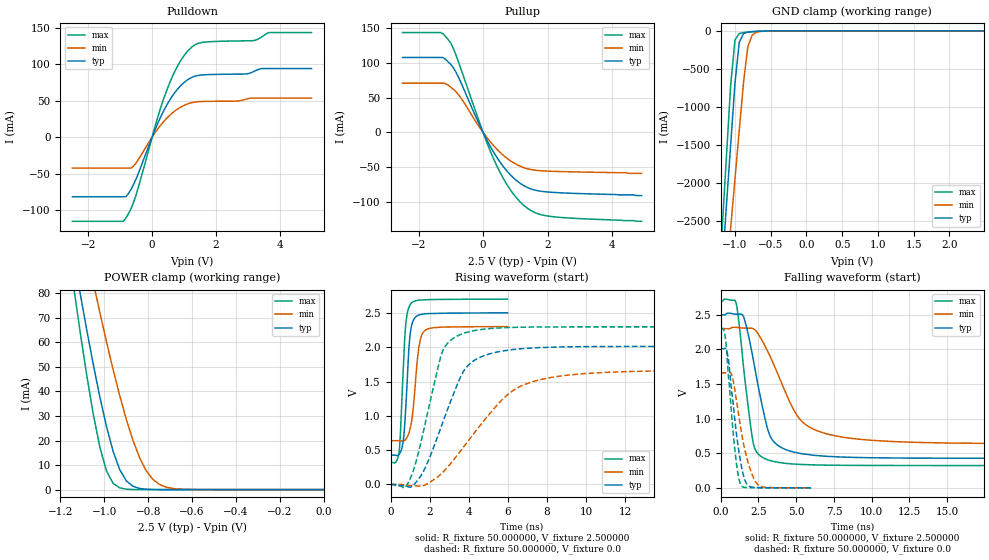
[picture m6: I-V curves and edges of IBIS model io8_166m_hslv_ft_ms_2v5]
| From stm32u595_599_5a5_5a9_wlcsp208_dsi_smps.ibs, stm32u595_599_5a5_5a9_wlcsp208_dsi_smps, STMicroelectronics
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|   Model io8_166m_hslv_ft_ms_2v5
[Model]  io8_166m_hslv_ft_ms_2v5
Model_type I/O
Polarity   Non-Inverting
Enable   Active-Low
Vinl =   0.750000V
Vinh =   1.750000V
Vmeas =  1.250000V
Cref =   50.000000pF
Rref =   100.000000M
Vref =   0.0V
C_comp   3.458600pF   3.458000pF   3.495600pF
[Temperature Range]   25.000000   0.140000k   -40.000000
[Pullup Reference]   2.500000V   2.300000V   2.700000V
[Pulldown Reference]   0.0V   0.0V   0.0V
[POWER Clamp Reference]   2.500000V   2.300000V   2.700000V
[GND Clamp Reference]   0.0V   0.0V   0.0V
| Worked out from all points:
|   slope of the pulldown table from 0 to 0.375 V, typ, clamps not added: 10.1 ohm
|   slope of the pullup table from 0 to 0.375 V, typ, clamps not added: 11.7 ohm
|   GND clamp passes 1 mA (typ) near -0.50 V on its own axis
|   POWER clamp passes 1 mA (typ) near -0.86 V on its own axis
|   rising waveform, R_fixture 50.000000, V_fixture 2.500000: 20-80 % time 251ps typ, 332ps min, 234ps max; typ from 0.428 V to 2.5 V
|   rising waveform, R_fixture 50.000000, V_fixture 0.0: 20-80 % time 1.64ns typ, 2.93ns min, 1.12ns max; typ from 0 V to 2.01 V
|   falling waveform, R_fixture 50.000000, V_fixture 2.500000: 20-80 % time 1.17ns typ, 2.21ns min, 750ps max; typ from 2.5 V to 0.428 V
|   falling waveform, R_fixture 50.000000, V_fixture 0.0: 20-80 % time 665ps typ, 867ps min, 543ps max; typ from 2.01 V to 0 V
[Pulldown]
|Voltage   I(typ)   I(min)   I(max)
-2.5V     -81.62mA   -42.31mA   -115.3mA
-900mV    -81.62mA   -42.31mA   -115.3mA
-820mV    -81.43mA   -42.31mA   -110.6mA
-500mV    -56.95mA   -35.08mA   -78.57mA
140mV     15.18mA    9.02mA     22.02mA
460mV     44mA       25.98mA    64.38mA
860mV     68.91mA    40.27mA    102.2mA
1.26V     82.21mA    47.42mA    124mA
1.66V     85.54mA    49mA       130.3mA
3.18V     89.84mA    53.64mA    132.3mA
3.66V     94.01mA    53.64mA    143.3mA
5V        94.01mA    53.64mA    143.3mA
[Pullup]
|Voltage   I(typ)   I(min)   I(max)
-2.5V     108.1mA    71.02mA    143.9mA
-1.32V    108.1mA    71.02mA    143.9mA
-1.24V    107.8mA    71.02mA    142.1mA
-1V       97.95mA    65.11mA    128.6mA
-680mV    71.17mA    49.12mA    90.46mA
-40mV     3.893mA    2.628mA    5.181mA
360mV     -30.97mA   -20.78mA   -41.56mA
840mV     -60.71mA   -40.52mA   -82.21mA
1.32V     -78.06mA   -51.54mA   -107.3mA
1.64V     -83.42mA   -54.54mA   -116.1mA
2.12V     -86.16mA   -55.91mA   -121.1mA
4.92V     -91mA      -59mA      -128mA
[GND_clamp]
|Voltage   I(typ)   I(min)   I(max)
-2.5V     -9.641A    -9.693A    -9.352A
-1.18V    -3.114A    -3.874A    -2.614A
-1.12V    -2.301A    -3.23A     -1.656A
-1.06V    -1.489A    -2.587A    -706.2mA
-1V       -685.8mA   -1.945A    -119.3mA
-940mV    -149.7mA   -1.304A    -34.73mA
-880mV    -35.54mA   -672.6mA   -23.06mA
-820mV    -16.2mA    -206.4mA   -17.27mA
-760mV    -10.58mA   -57.55mA   -12.41mA
-700mV    -7.152mA   -18.74mA   -8.24mA
-400mV    -103.3uA   -378.6uA   -41.75uA
2.48V     0A         13.22nA    0A
[POWER_clamp]
|Voltage   I(typ)   I(min)   I(max)
-2.49V    881mA      773.1mA    1.07A
-1.14V    95.25mA    122.7mA    82.82mA
-1.11V    79.9mA     109.7mA    64.14mA
-1.05V    50.87mA    84.26mA    30.57mA
-1.02V    37.63mA    72.04mA    17.17mA
-990mV    25.71mA    60.25mA    7.621mA
-930mV    8.217mA    38.43mA    713.9uA
-900mV    3.624mA    28.77mA    182.8uA
-840mV    490.7uA    13.24mA    11.35uA
-780mV    56.55uA    4.324mA    699nA
-660mV    716.7nA    226uA      9.784nA
0V        0A         19.53nA    0A
[Ramp]
| variable   typ   min   max
dV/dt_r  1.20666/1.63909n   0.99774/2.93063n   1.37784/1.11995n
dV/dt_f  1.24345/1.16615n   0.99710/2.20556n   1.42637/0.74900n
R_load = 50.000000
[Rising Waveform]
R_fixture= 50.000000
V_fixture= 2.500000
V_fixture_min= 2.300000
V_fixture_max= 2.700000
|time   V(typ)   V(min)   V(max)
0s        427.5mV    637.5mV    322.7mV
432.4ps   437mV      637.5mV    472.2mV
492.5ps   464.9mV    637.1mV    688.4mV
636.6ps   611.9mV    633.7mV    1.603V
792.8ps   1.202V     664mV      2.375V
924.9ps   1.922V     740.2mV    2.571V
1.021ns   2.228V     835.2mV    2.627V
1.441ns   2.468V     1.985V     2.685V
1.73ns    2.484V     2.235V     2.69V
5.982ns   2.5V       2.3V       2.7V
[Rising Waveform]
R_fixture= 50.000000
V_fixture= 0.0
V_fixture_min= 0.0
V_fixture_max= 0.0
|time   V(typ)   V(min)   V(max)
0s        -51.83uV   -11.86uV   11.83uV
800.8ps   -25.5mV    -13.53mV   -23.55mV
1.151ns   -13.85mV   -17.87mV   192.1mV
1.552ns   127.4mV    -23.34mV   613.3mV
2.653ns   891.1mV    172.7mV    1.935V
3.103ns   1.234V     316.9mV    2.107V
3.854ns   1.7V       591.6mV    2.213V
6.006ns   1.957V     1.314V     2.286V
8.158ns   1.999V     1.556V     2.295V
24.92ns   2.011V     1.663V     2.296V
[Falling Waveform]
R_fixture= 50.000000
V_fixture= 2.500000
V_fixture_min= 2.300000
V_fixture_max= 2.700000
|time   V(typ)   V(min)   V(max)
0s        2.5V       2.3V       2.7V
1.001ns   2.511V     2.32V      2.685V
1.502ns   2.478V     2.309V     1.767V
2.152ns   1.859V     2.3V       653.2mV
2.953ns   985.1mV    2.043V     419.5mV
3.554ns   657.7mV    1.762V     378.8mV
5.055ns   506.9mV    1.046V     341.4mV
6.757ns   460.1mV    797.2mV    329.2mV
11.46ns   431.6mV    668.5mV    323.2mV
24.92ns   427.5mV    637.5mV    322.7mV
[Falling Waveform]
R_fixture= 50.000000
V_fixture= 0.0
V_fixture_min= 0.0
V_fixture_max= 0.0
|time   V(typ)   V(min)   V(max)
0s        2.011V     1.663V     2.296V
288.3ps   2.018V     1.663V     2.198V
468.5ps   1.911V     1.663V     1.744V
720.7ps   1.405V     1.635V     1.067V
961ps     935.2mV    1.379V     503.4mV
1.153ns   602mV      1.109V     190.6mV
1.333ns   356.9mV    852.5mV    44.18mV
1.718ns   58.64mV    443.9mV    4.717mV
2.486ns   3.625mV    41.46mV    1.71mV
5.982ns   -51.83uV   -11.86uV   11.83uV
